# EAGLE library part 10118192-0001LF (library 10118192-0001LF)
Micro USB, Input Output Connectors, B TYPE RECEPTACLE with flange Source: Datasheet
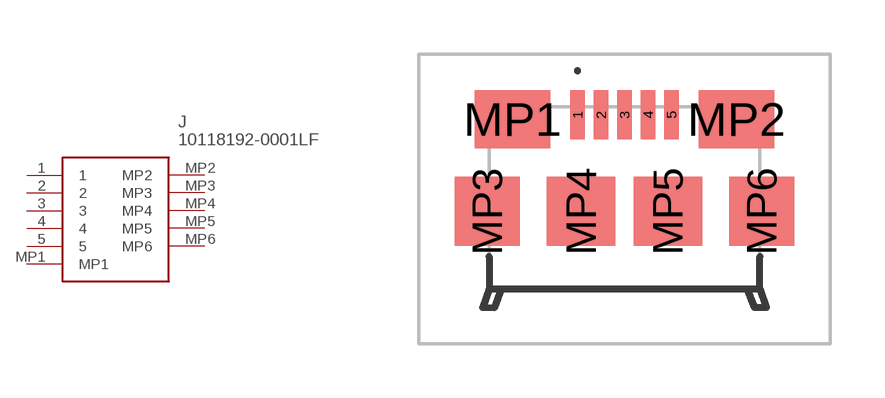
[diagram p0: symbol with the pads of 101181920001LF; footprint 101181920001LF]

Designator prefix J

## 10118192-0001LF (Arrow_Part_Number: 10118192-0001LF; Arrow_Price-Stock: https://www.arrow.com/en/products/10118192-0001lf/amphenol-fci?region=nac; Description: Micro USB, Input Output Connectors, B TYPE RECEPTACLE with flange; Height: 3.05mm; Manufacturer_Name: Amphenol Communications Solutions; Manufacturer_Part_Number: 10118192-0001LF)  [101181920001LF]
1  1
2  2
3  3
4  4
5  5
MP1  MP1
MP2  MP2
MP3  MP3
MP4  MP4
MP5  MP5
MP6  MP6

## Footprint 101181920001LF (pad centres in mm)
10118192-0001LF-4
smd 0.4 x 1.35: 1 -1.3,2.335; 2 -0.65,2.335; 3 0,2.335; 4 0.65,2.335; 5 1.3,2.335
smd 2.1 x 1.6: MP1 -3.1,2.21; MP2 3.1,2.21
smd 1.8 x 1.9: MP3 -3.8,-0.34; MP6 3.8,-0.34
smd 1.9 x 1.9: MP4 -1.2,-0.34; MP5 1.2,-0.34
